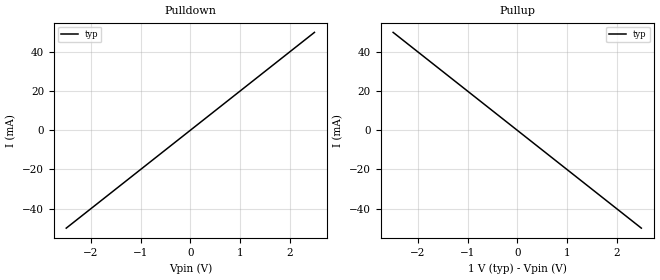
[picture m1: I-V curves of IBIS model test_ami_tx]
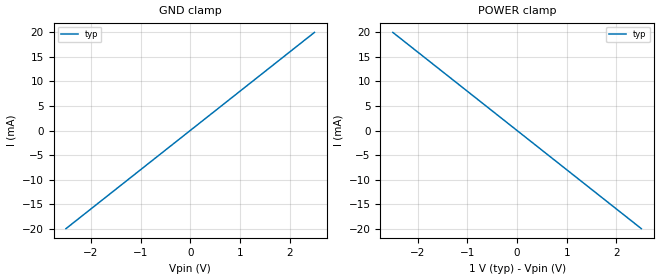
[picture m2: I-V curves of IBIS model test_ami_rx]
|   TEST IBIS-AMI Models
[IBIS Ver]   5.0
[Disclaimer]
   THIS IBIS MODEL IS PROVIDED "AS IS" AND WITH NO
   WARRANTIES, INCLUDING WITHOUT LIMITATION ANY EXPRESS
   WARRANTIES OR IMPLIED WARRANTIES OF MERCHANTABILITY
   OR FITNESS FOR A PARTICULAR USE. THIS MODEL IS CREATED
   TO BE USED FOR TEST PURPOSES ALONG WITH AMI MODELS.
[File Name]  test_ibis.ibs
[Date]   March 25, 2010
[File Rev]   1.0
[Source]   Cadence Design System
[Notes]   Revision 1.0 -- 03/25/2010
[Copyright]  Copyright 2010, Cadence Design System.,
   All Rights Reserved.
|   COMPONENT: test_serdes
[Component] test_serdes
[Manufacturer]  CDNS
[Package]
R_pkg   0.01m  NA NA
L_pkg   0.01nH NA NA
C_pkg   0.01pF NA NA
[Pin] signal_name   model_name   R_pin L_pin C_pin
1   ami_tx_p   test_ami_tx   NA   NA   NA
2   ami_tx_n   test_ami_tx   NA   NA   NA
3   ami_rx_p   test_ami_rx   NA   NA   NA
4   ami_rx_n   test_ami_rx   NA   NA   NA
[Diff Pin] inv_pin  vdiff tdelay_typ tdelay_min tdelay_max
1   2   0.01V   NA   NA   NA
3   4   0.01V   NA   NA   NA
| Models and submodels in the file (2): test_ami_tx (Output), test_ami_rx (Input)
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|   MODEL: test_ami_tx
[Model]   test_ami_tx
Model_type Output
Vmeas = .1
|   typ   min   max
C_comp   0.2pF 0.2pF 0.2pF
[Algorithmic Model]
Executable i86_VS_32 IBIS_AMI_CHGAIN.dll   IBIS_AMI_CHGAIN.ami
|Executable Linux_gcc4.1.2_32   IBIS_AMI_CHGAIN.dll   IBIS_AMI_CHGAIN.ami
[End Algorithmic Model]
[Voltage Range]   1.0  1.0  1.0
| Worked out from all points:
|   slope of the pulldown table from 0 to 0.15 V, typ, clamps not added: 50 ohm
|   slope of the pullup table from 0 to 0.15 V, typ, clamps not added: 50 ohm
[Pulldown]
-2.5V     -50mA      NA         NA
0V        0A         NA         NA
2.5V      50mA       NA         NA
[Pullup]
-2.5V     50mA       NA         NA
0V        0A         NA         NA
2.5V      -50mA      NA         NA
[Ramp]
dV/dt_r 0.2/20p 0.2/20p 0.2/20p
dV/dt_f 0.2/20p 0.2/20p 0.2/20p
|   MODEL: test_ami_rx
[Model]   test_ami_rx
Model_type Input
Vinl = .5
Vinh = .5
|   typ   min   max
C_comp   0.4pF 0.4pF 0.4pF
[Algorithmic Model]
Executable i86_VS_32 IBIS_AMI_RX_CTF.dll   IBIS_AMI_RX_CTF.ami
|Executable Linux_gcc4.1.2_32   IBIS_AMI_RX_CTF.so   IBIS_AMI_RX_CTF.ami
[End Algorithmic Model]
[Temperature Range]  25   100  0
[Voltage Range]   1.0  1.0  1.0
[GND Clamp]
-2.5V     -20mA      NA         NA
0V        0A         NA         NA
2.5V      20mA       NA         NA
[Power Clamp]
-2.5V     20mA       NA         NA
0V        0A         NA         NA
2.5V      -20mA      NA         NA
